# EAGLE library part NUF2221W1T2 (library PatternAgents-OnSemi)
NUF2221W1T2 USB ESD Protection, EMI FIlter, and Line Termination
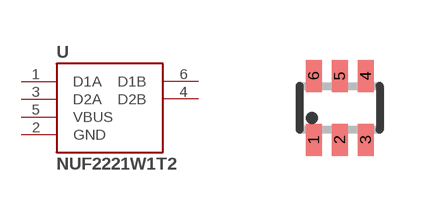
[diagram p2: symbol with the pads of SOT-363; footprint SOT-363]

Designator prefix -

## NUF2221W1T2  [SOT-363]
1  D1A
2  GND
3  D2A
4  D2B
5  VBUS
6  D1B

## Footprint SOT-363 (pad centres in mm)
SOT-363 Small Outline Transistor; 6 leads
smd 0.4 x 0.8: 1 -0.65,-0.8; 2 0,-0.8; 3 0.65,-0.8; 4 0.65,0.8; 5 0,0.8; 6 -0.65,0.8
